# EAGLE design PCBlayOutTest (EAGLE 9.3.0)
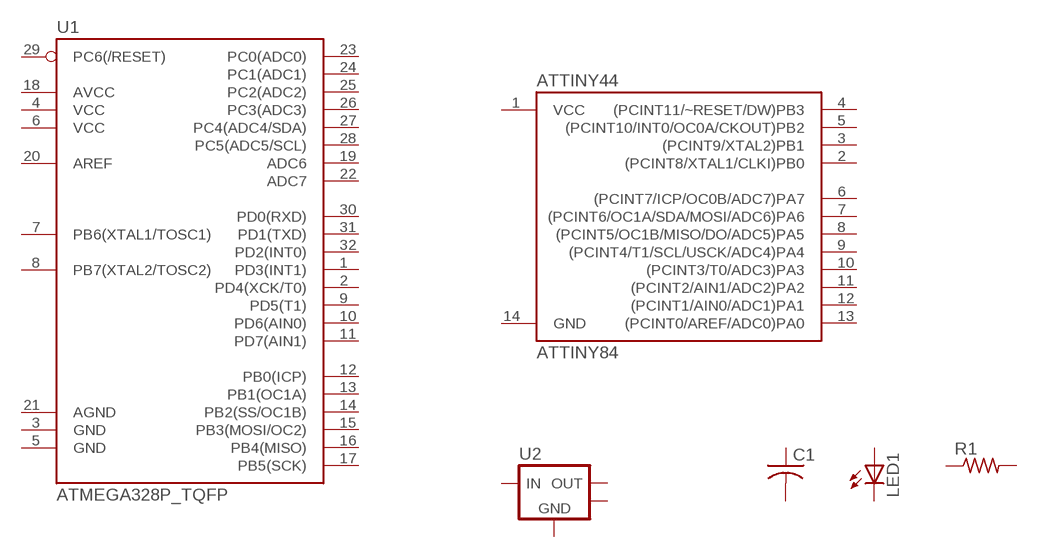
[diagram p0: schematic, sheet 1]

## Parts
ATTINY44  ATTINY84  [SO14]
C1  C-USC1206  [C1206]
LED1  LEDCHIPLED_1206  [CHIPLED_1206]
R1  R-US_M1206  [M1206]
U1  ATMEGA328P_TQFP  [TQFP32-08]
U2  LM2940DCY  [SOT-223-3]
Unconnected: ATTINY44.1(VCC) ATTINY44.2((PCINT8/XTAL1/CLKI)PB0) ATTINY44.3((PCINT9/XTAL2)PB1) ATTINY44.4((PCINT11/~RESET/DW)PB3) ATTINY44.5((PCINT10/INT0/OC0A/CKOUT)PB2) ATTINY44.6((PCINT7/ICP/OC0B/ADC7)PA7) ATTINY44.7((PCINT6/OC1A/SDA/MOSI/ADC6)PA6) ATTINY44.8((PCINT5/OC1B/MISO/DO/ADC5)PA5) ATTINY44.9((PCINT4/T1/SCL/USCK/ADC4)PA4) ATTINY44.10((PCINT3/T0/ADC3)PA3) ATTINY44.11((PCINT2/AIN1/ADC2)PA2) ATTINY44.12((PCINT1/AIN0/ADC1)PA1) ATTINY44.13((PCINT0/AREF/ADC0)PA0) ATTINY44.14(GND) C1.1 C1.2 LED1.A LED1.C R1.1 R1.2 U1.1(PD3(INT1)) U1.2(PD4(XCK/T0)) U1.3(GND) U1.4(VCC) U1.5(GND) U1.6(VCC) U1.7(PB6(XTAL1/TOSC1)) U1.8(PB7(XTAL2/TOSC2)) U1.9(PD5(T1)) U1.10(PD6(AIN0)) U1.11(PD7(AIN1)) U1.12(PB0(ICP)) U1.13(PB1(OC1A)) U1.14(PB2(SS/OC1B)) U1.15(PB3(MOSI/OC2)) U1.16(PB4(MISO)) U1.17(PB5(SCK)) U1.18(AVCC) U1.19(ADC6) U1.20(AREF) U1.21(AGND) U1.22(ADC7) U1.23(PC0(ADC0)) U1.24(PC1(ADC1)) U1.25(PC2(ADC2)) U1.26(PC3(ADC3)) U1.27(PC4(ADC4/SDA)) U1.28(PC5(ADC5/SCL)) U1.29(PC6(/RESET)) U1.30(PD0(RXD)) U1.31(PD1(TXD)) U1.32(PD2(INT0)) U2.2(GND) U2.4(TAB)

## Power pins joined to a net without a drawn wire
VIN: U2.1(VIN)
VOUT: U2.3(VOUT)

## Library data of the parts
ATTINY44 = SparkFun-IC-Microcontroller:ATTINY84: Atmel 14-pin 2/4/8kB flash uC Datasheet SparkFun Products Tiny AVR Programmer (PGM-11801) SparkFun Servo Trigger - Continuous Rotation (WIG-13872) SparkFun Servo Trigger (WIG-13118); PROD_ID: IC-11285
C1 = adafruit:C-US: CAPACITOR, American symbol
LED1 = adafruit:LED: LED
R1 = adafruit:R-US_: RESISTOR, American symbol
U1 = SparkFun-IC-Microcontroller:ATMEGA328P_TQFP: Popular 328P in QFP Storefront component: ATmega328 - TQFP (COM-13448) Datasheet SparkFun Products SparkFun RedBoard - Programmed with Arduino (DEV-12757) Arduino Pro Mini 328 - 5V/16MHz (DEV-11113) Arduino Pro Mini 328 - 3.3V/8MHz (DEV-11114) SparkFun OpenLog (DEV-13712) SparkFun MicroView - OLED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; PROD_ID: IC-09069
U2 = bt_regulator:LM2940: LM2940 LDO Voltage Regulator Input Voltage Range = 6 V to 26 V Dropout Voltage Typically 0.5 V at IOUT = 1 A Reverse Battery Protection Internal Short Circuit Current Limit electrostatic discharge protection (±2kV) Tab is GND The LM2940-N/LM2940C positive voltage regulator features the ability to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

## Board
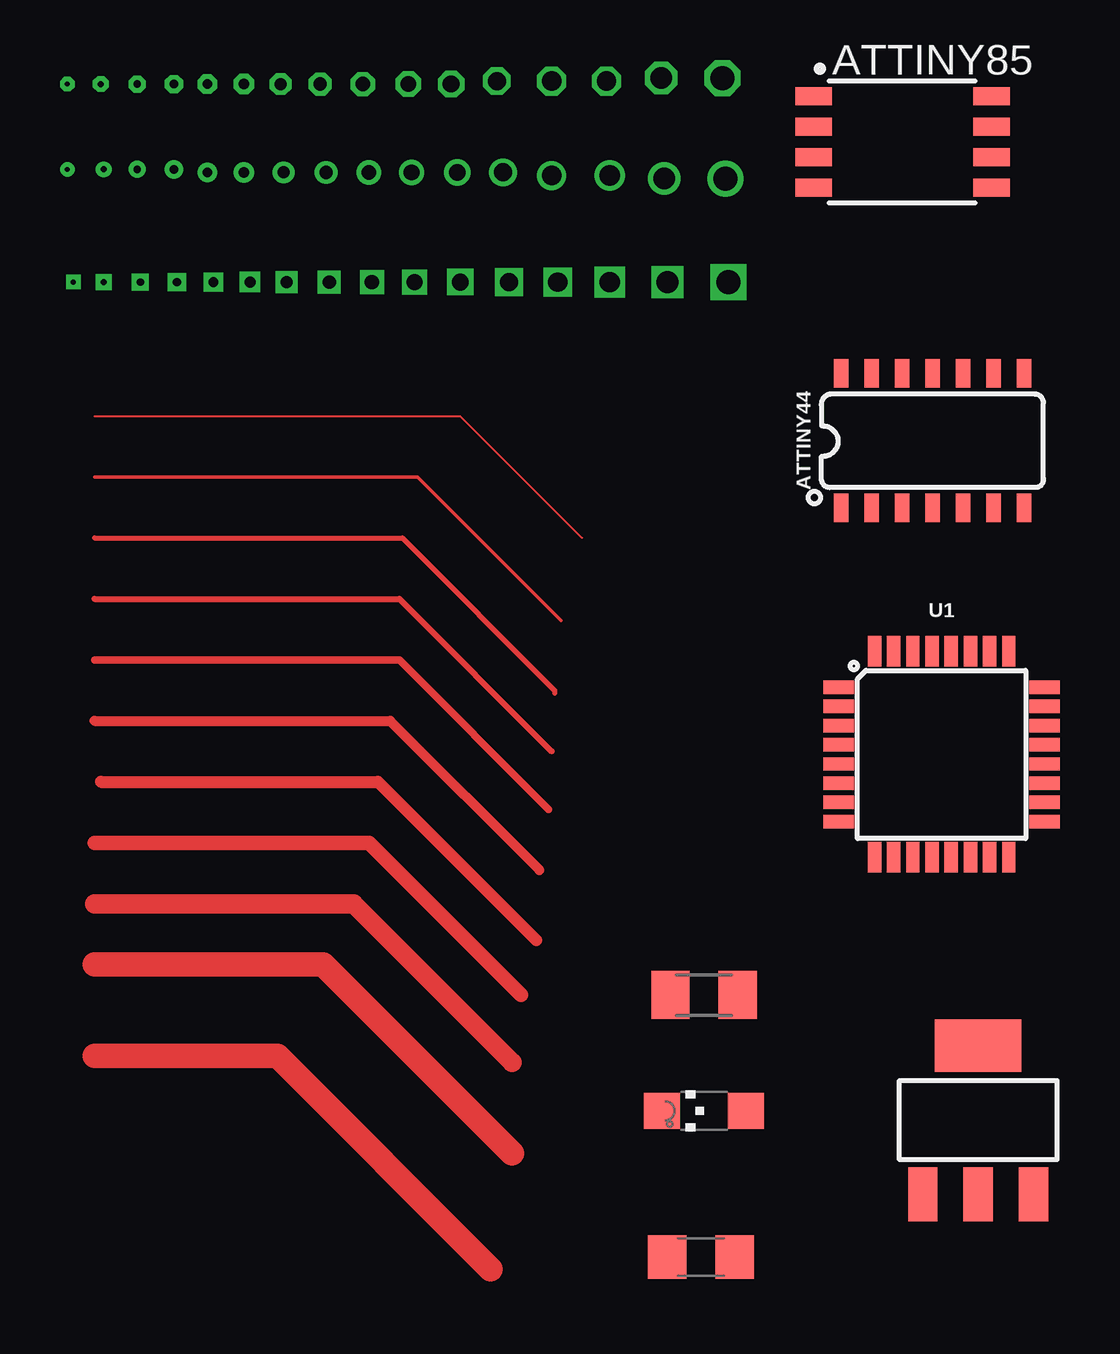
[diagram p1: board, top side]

No outline drawn. Coordinates in mm, seen from the top.
Copper layers (1*16): Top 0.035mm / dielectric 1.5mm / Bottom 0.035mm
Design rules "default": minimum track width 6mil, minimum drill 0.35mm, track to track 6mil, track to pad 6mil, pad to pad 6mil, via to via 6mil, smd to smd 6mil, copper to edge 40mil, drill to drill 6mil, minimum pad ring 10mil, minimum via ring 8mil, stop-mask expansion 4mil, vias tented up to drill 0mil, thermal gap 10mil

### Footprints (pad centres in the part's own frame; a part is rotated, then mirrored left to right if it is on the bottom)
SO14 = smd 0.6 x 1.2: 1 -3.175,-2.8; 2 -1.905,-2.8; 3 -0.635,-2.8; 4 0.635,-2.8; 5 1.905,-2.8; 6 3.175,-2.8; 7 4.445,-2.8; 8 4.445,2.8; 9 3.175,2.8; 10 1.905,2.8; 11 0.635,2.8; 12 -0.635,2.8; 13 -1.905,2.8; 14 -3.175,2.8
ATTINY85 = smd 1.524 x 0.762: 1 -3.683,1.905; 2 -3.683,0.635; 3 -3.683,-0.635; 4 -3.683,-1.905; 5 3.727,-1.905; 6 3.727,-0.635; 7 3.727,0.635; 8 3.727,1.905
C1206 = smd 1.6 x 1.8: 1 -1.4,0; 2 1.4,0
CHIPLED_1206 = smd 1.5 x 1.5: A 0,-1.75; C 0,1.75
M1206 = smd 1.6 x 2: 1 -1.4,0; 2 1.4,0
TQFP32-08 = smd 1.27 x 0.559: 1 -4.293,2.8; 2 -4.293,2; 3 -4.293,1.2; 4 -4.293,0.4; 5 -4.293,-0.4; 6 -4.293,-1.2; 7 -4.293,-2; 8 -4.293,-2.8; 17 4.293,-2.8; 18 4.293,-2; 19 4.293,-1.2; 20 4.293,-0.4; 21 4.293,0.4; 22 4.293,1.2; 23 4.293,2; 24 4.293,2.8 | smd 0.559 x 1.27: 9 -2.8,-4.293; 10 -2,-4.293; 11 -1.2,-4.293; 12 -0.4,-4.293; 13 0.4,-4.293; 14 1.2,-4.293; 15 2,-4.293; 16 2.8,-4.293; 25 2.8,4.293; 26 2,4.293; 27 1.2,4.293; 28 0.4,4.293; 29 -0.4,4.293; 30 -1.2,4.293; 31 -2,4.293; 32 -2.8,4.293
SOT-223-3 = smd 1.219 x 2.235: 1 -2.311,-3.099; 2 0,-3.099; 3 2.311,-3.099 | smd 3.6 x 2.2: 4 0,3.099

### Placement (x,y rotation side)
ATTINY44  35.56,-12.45 0 top
ATTINY85  [ATTINY85]  34.92,0 0 top
C1  26.54,-46.48 0 top
LED1  26.67,-40.39 90 top
R1  26.67,-35.56 0 top
U1  36.58,-25.53 0 top
U2  38.1,-40.77 0 top

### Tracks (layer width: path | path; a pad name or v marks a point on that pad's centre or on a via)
D  (via drill 0.8)
  other vias: 20.32,2.54
S$1  (via drill 0.2)
  other vias: 0.13,-1.14
S$2  (via drill 0.25)
  other vias: 1.65,-1.14
S$3  (via drill 0.3)
  other vias: 3.05,-1.14
S$4  (via drill 0.35)
  other vias: 4.57,-1.14
S$5  (via drill 0.4)
  other vias: 5.97,-1.27
S$6  (via drill 0.45)
  other vias: 7.49,-1.27
S$7  (via drill 0.5)
  other vias: 9.14,-1.27
S$8  (via drill 0.55)
  other vias: 10.92,-1.27
S$9  (via drill 0.6)
  other vias: 12.7,-1.27
S$10  (via drill 0.65)
  other vias: 14.48,-1.27
S$11  (via drill 0.7)
  other vias: 16.38,-1.27
S$12  (via drill 0.75)
  other vias: 18.29,-1.27
S$13  (via drill 0.8)
  other vias: 20.32,-1.4
S$14  (via drill 0.85)
  other vias: 22.73,-1.4
S$15  (via drill 0.9)
  other vias: 25.02,-1.52
S$16  (via drill 1)
  other vias: 27.56,-1.52
S$17  (via drill 1)
  other vias: 27.69,-5.84
S$18  (via drill 0.9)
  other vias: 25.15,-5.84
S$19  (via drill 0.85)
  other vias: 22.73,-5.84
S$20  (via drill 0.8)
  other vias: 20.57,-5.84
S$21  (via drill 0.75)
  other vias: 18.54,-5.84
S$22  (via drill 0.7)
  other vias: 16.51,-5.84
S$23  (via drill 0.65)
  other vias: 14.61,-5.84
S$24  (via drill 0.6)
  other vias: 12.83,-5.84
S$25  (via drill 0.55)
  other vias: 11.05,-5.84
S$26  (via drill 0.5)
  other vias: 9.27,-5.84
S$27  (via drill 0.45)
  other vias: 7.75,-5.84
S$28  (via drill 0.4)
  other vias: 6.22,-5.84
S$29  (via drill 0.35)
  other vias: 4.7,-5.84
S$30  (via drill 0.3)
  other vias: 3.17,-5.84
S$31  (via drill 0.25)
  other vias: 1.65,-5.84
S$32  (via drill 0.2)
  other vias: 0.38,-5.84
S$33  (via drill 0.2)
  other vias: 0.13,2.41
S$34  (via drill 0.25)
  other vias: 1.52,2.41
S$35  (via drill 0.3)
  other vias: 3.05,2.41
S$36  (via drill 0.35)
  other vias: 4.57,2.41
S$37  (via drill 0.4)
  other vias: 5.97,2.41
S$38  (via drill 0.45)
  other vias: 7.49,2.41
S$39  (via drill 0.5)
  other vias: 9.02,2.41
S$40  (via drill 0.55)
  other vias: 10.67,2.41
S$41  (via drill 0.6)
  other vias: 12.45,2.41
S$42  (via drill 0.65)
  other vias: 14.35,2.41
S$43  (via drill 0.7)
  other vias: 16.13,2.41
S$44  (via drill 0.75)
  other vias: 18.03,2.54
S$45  (via drill 0.8)
  other vias: 22.61,2.54
S$46  (via drill 0.9)
  other vias: 24.89,2.67
S$47  (via drill 1)
  other vias: 27.43,2.67
S$49
  Top 0.076: 1.27,-11.43 16.51,-11.43 21.59,-16.51
S$50
  Top 0.152: 1.27,-13.97 14.73,-13.97 20.7,-19.94
S$51
  Top 0.203: 1.27,-16.51 14.1,-16.51 20.45,-22.86 20.45,-22.99
S$52
  Top 0.254: 1.27,-19.05 13.97,-19.05 20.32,-25.4
S$53
  Top 0.305: 1.27,-21.59 13.97,-21.59 20.19,-27.81
S$54
  Top 0.406: 1.27,-24.13 13.59,-24.13 19.81,-30.35
S$55
  Top 0.508: 1.52,-26.67 13.08,-26.67 19.68,-33.27
S$56
  Top 0.61: 1.27,-29.21 12.7,-29.21 19.05,-35.56
S$57
  Top 0.813: 1.27,-31.75 12.06,-31.75 18.67,-38.35
S$58
  Top 1.016: 1.27,-34.29 10.79,-34.29 18.67,-42.16
S$59
  Top 1.016: 1.27,-38.1 8.89,-38.1 17.78,-46.99

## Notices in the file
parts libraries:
SparkFun-IC-Microcontroller: Licensing: Creative Commons ShareAlike 4.0 International - https://creativecommons.org/licenses/by-sa/4.0
